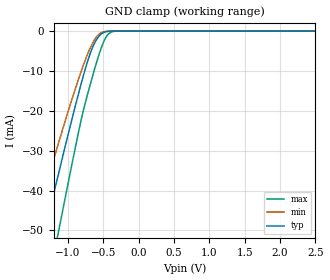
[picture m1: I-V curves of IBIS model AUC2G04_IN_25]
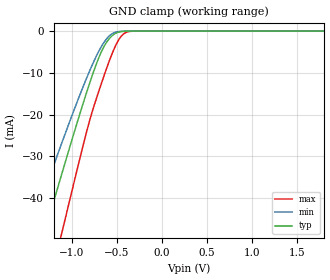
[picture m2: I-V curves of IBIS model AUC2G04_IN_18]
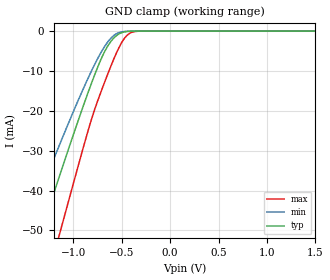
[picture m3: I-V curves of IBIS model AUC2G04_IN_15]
| TEXAS INSTRUMENTS INCORPORATED
| Standard Linear and Logic Group
| IBIS Model of SN74AUC2G04
| DUAL INVERTER GATE
| This file contains package information for the following:
|  SOT 6-pin (DBV) package as [Component] AUC2G04_DBV
|  SOT 6-pin (DCK) package as [Component] AUC2G04_DCK
|  NanoStar WCSP 6-pin (YEA) package as [Component] AUG2G04_YEA
|  NanoFree WCSP 6-pin (YZA) package as [Component] AUC2G04_YZA
| This device can be powered at the following Vccs:
|  2.5 volt Vcc
|  1.8 volt Vcc
|  1.5 volt Vcc
|  1.2 volt Vcc
|  0.8 volt Vcc
| This file provides unique models under the [Model Selector] for each Vcc.
| For operation at a specific Vcc, select the appropriate model after each
| [Model Selector] keyword.
[IBIS Ver]   3.2
[Comment char]  |_char
[File Name]   sn74auc2g04.ibs
[File Rev]   1.2 | x_die
[Date]   September 16, 2003
[Source]   Data created from TI-SPICE simulations at TI-SLL.
[Notes]   The following is an IBIS list for the SN74AUC2G04.
   Please contact sllibis@ti.com with questions and
   comments concerning SLL IBIS models.
   - Power-clamp data has been deleted since there is no
   power-clamp diode in the device.
   - Non-monotonic data in pullup and pulldown due to feedback
   circuit.
[Disclaimer] Property of Texas Instruments Incorporated. Unauthorized
   reproduction and/or distribution is strictly prohibited.
   This product is protected under copyright law.
   Created 2002,(C) Copyright 2002, Texas Instruments
   Incorporated, All Rights Reserved
   UNLESS THERE IS A SIGNED, WRITTEN AGREEMENT TO THE
   CONTRARY, TEXAS INSTRUMENTS (TI) IS PROVIDING THE IBIS
   MODELS AND WITHOUT ANY WARRANTY, EXPRESSED OR
   IMPLIED. TI assumes no liability for:
   1) the accuracy of the IBIS models provided to your
   company;
   2) the proper functioning of these IBIS Models in your
   design or for any resulting applications; or
   3) infringement of patents, copyrights or intellectual
   property rights resulting from your use of these IBIS
   models.
   TI provides IBIS Models as a service to our customers.
   You and your company shall not distribute, sell or give
   these models to anyone else without prior written
   permission from TI.
   TI reserves the right to make changes to our products or
   to discontinue any semiconductor product or service
   without notice, and advises our customers to obtain the
   latest version of relevant information to verify, before
   placing orders, that the information being relied on is
   current.
   Please be aware that your receipt and use of the IBIS
   information provided shall serve as acceptance of these
   terms and conditions. If you do not accept these terms,
   you should return or destroy the IBIS models and any
   other accompanying information immediately.
| Component AUC2G04_DBV 6-pin SOT
[Component]   AUC2G04_DBV
[Manufacturer]   Texas Instruments, Inc.
[Package]
|   typ   min   max
R_pkg   0.025   0.019   0.037
L_pkg   1.524nH   1.260nH   1.751nH
C_pkg   0.245pF   0.198pF   0.264pF
[Pin]   signal_name   model_name   R_pin   L_pin   C_pin
1   1A   AUC2G04_IN   0.021   1.405nH   0.246pF
2   GND   GND   0.037   1.751nH   0.263pF
3   2A   AUC2G04_IN   0.026   1.493nH   0.247pF
4   2Y   AUC2G04_OUT   0.019   1.620nH   0.264pF
5   VCC   POWER   0.024   1.260nH   0.198pF
6   1Y   AUC2G04_OUT   0.021   1.617nH   0.250pF
| Component AUC2G04_DCK 6-pin SOT
[Component]   AUC2G04_DCK
[Manufacturer]   Texas Instruments, Inc.
[Package]
|   typ   min   max
R_pkg   1.400e-02   1.100e-02   2.100e-02
L_pkg   9.480e-10   7.840e-10   1.103e-09
C_pkg   1.910e-13   1.670e-13   2.050e-13
[Pin]   signal_name   model_name   R_pin   L_pin   C_pin
1   1A   AUC2G04_IN   1.300e-02   9.840e-10   1.960e-13
2   GND   GND   2.100e-02   1.103e-09   2.050e-13
3   2A   AUC2G04_IN   1.100e-02   9.980e-10   1.970e-13
4   2Y   AUC2G04_OUT   1.300e-02   9.040e-10   1.900e-13
5   VCC   POWER   1.500e-02   7.840e-10   1.670e-13
6   1Y   AUC2G04_OUT   1.200e-02   9.160e-10   1.950e-13
| Component AUC2G04_YEA 6-pin NanoStar WCSP
[Component]   AUC2G04_YEA
[Manufacturer]   Texas Instruments, Inc.
[Package]
|   typ   min   max
R_pkg   0.001   0.001   0.001
L_pkg   1.021nH   1.021nH   1.021nH
C_pkg   0.047pF   0.046pF   0.047pF
[Pin]   signal_name   model_name   R_pin   L_pin   C_pin
1   1A   AUC2G04_IN   0.001   0.021nH   0.046pF
2   GND   GND   0.001   0.021nH   0.047pF
3   2A   AUC2G04_IN   0.001   0.021nH   0.046pF
4   2Y   AUC2G04_OUT   0.001   0.021nH   0.046pF
5   VCC   POWER   0.001   0.021nH   0.047pF
6   1Y   AUC2G04_OUT   0.001   0.021nH   0.046pF
| Component AUC2G04_YZA 6-pin NanoFree WCSP
[Component]   AUC2G04_YZA
[Manufacturer]   Texas Instruments, Inc.
[Package]
|   typ   min   max
R_pkg   0.001   0.001   0.001
L_pkg   1.021nH   1.021nH   1.021nH
C_pkg   0.047pF   0.046pF   0.047pF
[Pin]   signal_name   model_name   R_pin   L_pin   C_pin
1   1A   AUC2G04_IN   0.001   0.021nH   0.046pF
2   GND   GND   0.001   0.021nH   0.047pF
3   2A   AUC2G04_IN   0.001   0.021nH   0.046pF
4   2Y   AUC2G04_OUT   0.001   0.021nH   0.046pF
5   VCC   POWER   0.001   0.021nH   0.047pF
6   1Y   AUC2G04_OUT   0.001   0.021nH   0.046pF
| Model AUC2G04_IN
[Model Selector]   AUC2G04_IN
AUC2G04_IN_25   2.5 volt Vcc
AUC2G04_IN_18   1.8 volt Vcc
AUC2G04_IN_15   1.5 volt Vcc
AUC2G04_IN_12   1.2 volt Vcc
AUC2G04_IN_08   0.8 volt Vcc
| Model AUC2G04_OUT
[Model Selector]   AUC2G04_OUT
AUC2G04_OUT_25   2.5 volt Vcc
AUC2G04_OUT_18   1.8 volt Vcc
AUC2G04_OUT_15   1.5 volt Vcc
AUC2G04_OUT_12   1.2 volt Vcc
AUC2G04_OUT_08   0.8 volt Vcc
| Models and submodels in the file (10): AUC2G04_IN_25 (Input), AUC2G04_IN_18 (Input), AUC2G04_IN_15 (Input), AUC2G04_IN_12 (Input), AUC2G04_IN_08 (Input), AUC2G04_OUT_25 (Output), AUC2G04_OUT_18 (Output), AUC2G04_OUT_15 (Output), AUC2G04_OUT_12 (Output), AUC2G04_OUT_08 (Output)
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[Model]   AUC2G04_IN_25
Model_type  Input
Vinl=0.7
Vinh=1.7
| variable   typ   min   max
C_comp   2.28pF   1.82pF   2.66pF
[Temperature Range]   40   100   -40
| Ambient temperature   25   85   -40
[Voltage range]   2.5   2.3   2.7
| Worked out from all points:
|   GND clamp passes 1 mA (typ) near -0.55 V on its own axis
[GND Clamp]
| AUC2G04_IN_25
|   Voltage   I(typ)   I(min)   I(max)
-3.6V     -222.3mA   -186.1mA   -267.5mA
-1.49V    -62.29mA   -49.79mA   -82.1mA
-1.35V    -51.8mA    -41.14mA   -69.63mA
-1.305V   -48.45mA   -38.39mA   -65.61mA
-1.17V    -38.46mA   -30.25mA   -53.55mA
-1.12V    -34.79mA   -27.28mA   -49.08mA
-735mV    -8.324mA   -6.331mA   -16.67mA
-635mV    -3.426mA   -2.471mA   -10.25mA
-525mV    -682.5uA   -360.4uA   -4.021mA
-430mV    -73.19uA   -34.73uA   -776.9uA
-325mV    -3.339uA   -2.006uA   -30.74uA
2.5V      313.9pA    400.9pA    470.4pA
[Model]   AUC2G04_IN_18
Model_type  Input
Vinl=0.5775
Vinh=1.2675
| variable   typ   min   max
C_comp   2.35pF   1.91pF   2.66pF
[Temperature Range]   40   100   -40
| Ambient temperature   25   85   -40
[Voltage range]   1.8   1.65   1.95
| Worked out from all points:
|   GND clamp passes 1 mA (typ) near -0.55 V on its own axis
[GND Clamp]
| AUC2G04_IN_18
|   Voltage   I(typ)   I(min)   I(max)
-3.6V     -222.3mA   -186.1mA   -267.5mA
-1.475V   -61.16mA   -48.85mA   -80.77mA
-1.43V    -57.79mA   -46.07mA   -76.76mA
-1.295V   -47.7mA    -37.79mA   -64.71mA
-1.145V   -36.62mA   -28.76mA   -51.31mA
-1.095V   -32.97mA   -25.81mA   -46.85mA
-830mV    -14.31mA   -10.96mA   -23.64mA
-685mV    -5.607mA   -4.224mA   -13.41mA
-560mV    -1.272mA   -753.7uA   -5.827mA
-485mV    -290.6uA   -140.2uA   -2.305mA
-420mV    -55.81uA   -26.72uA   -608.5uA
1.8V      203.2pA    297.2pA    235.5pA
[Model]   AUC2G04_IN_15
Model_type  Input
Vinl=0.49
Vinh=1.04
| variable   typ   min   max
C_comp   2.39pF   1.96pF   2.69pF
[Temperature Range]   40   100   -40
| Ambient temperature   25   85   -40
[Voltage range]   1.5   1.4   1.6
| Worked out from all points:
|   GND clamp passes 1 mA (typ) near -0.55 V on its own axis
[GND Clamp]
| AUC2G04_IN_15
|   Voltage   I(typ)   I(min)   I(max)
-3.6V     -222.3mA   -186.1mA   -267.5mA
-1.505V   -63.42mA   -50.72mA   -83.44mA
-1.325V   -49.94mA   -39.61mA   -67.39mA
-1.17V    -38.46mA   -30.25mA   -53.55mA
-1.12V    -34.79mA   -27.28mA   -49.08mA
-840mV    -14.98mA   -11.48mA   -24.46mA
-695mV    -6.114mA   -4.621mA   -14.06mA
-570mV    -1.487mA   -911.6uA   -6.381mA
-495mV    -364.6uA   -178.8uA   -2.692mA
-430mV    -73.19uA   -34.73uA   -776.9uA
-280mV    -781.4nA   -556.3nA   -5.358uA
1.5V      165.9pA    258.5pA    172.1pA
